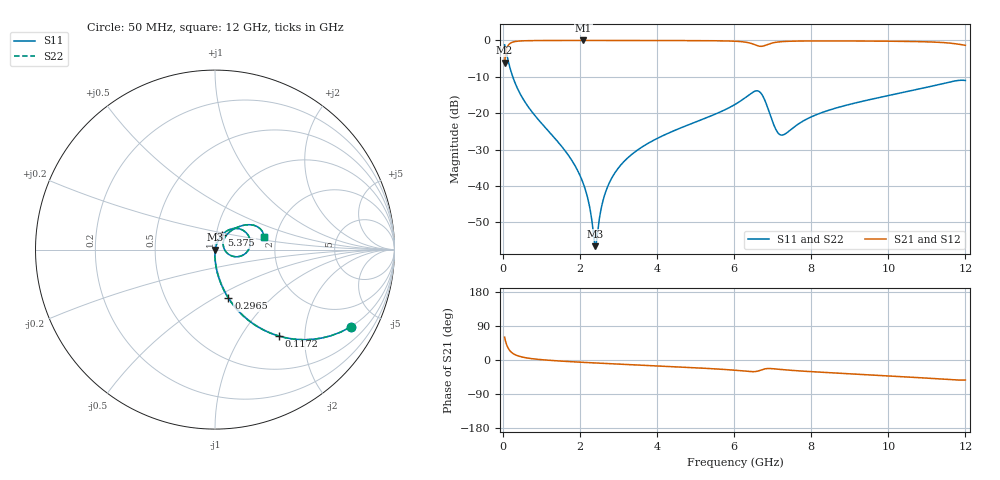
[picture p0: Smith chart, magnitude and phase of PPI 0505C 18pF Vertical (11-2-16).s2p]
# GHz S MA R 50
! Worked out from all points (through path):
!   1601 points, 50 MHz to 12 GHz, reference 50 ohm
!   highest |S21| = -0.01 dB at 2.089 GHz (marker M1); lowest = -6.1 dB at 50 MHz (marker M2)
!   group delay of S21, straight-line fit = 13.9 ps
!   lowest |S11| = -56.6 dB at 2.403 GHz (marker M3), VSWR 1.00, Z = 50.1 - j0.0292 ohm
!   |S11| at or under -10 dB: 261.2 MHz to end of sweep
!   |S22| runs from -56.6 to -1.2 dB; largest |S21 - S12| = 0
!   S11 on the Smith chart (normalised r, x): 50 MHz: 0.99, -3.51; 117.2 MHz: 0.99, -1.49; 296.5 MHz: 0.99, -0.58; 5.375 GHz: 1.07, +0.18; 12 GHz: 1.72, +0.26
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0.05  0.8696 -29.7  0.4937 60.2  0.4937 60.2  0.8696 -29.7
0.1172187  0.5998 -53.5  0.7998 36.5  0.7998 36.5  0.5998 -53.5
0.1919063  0.415 -66.0  0.9094 23.9  0.9094 23.9  0.415 -66.0
0.2964688  0.2809 -74.5  0.9592 15.3  0.9592 15.3  0.2809 -74.5
0.8043438  0.09723 -86.5  0.9943 2.9  0.9943 2.9  0.09723 -86.5
1.655781  0.02858 -91.3  0.9983 -3.8  0.9983 -3.8  0.02858 -91.3
2.044156  0.01243 -89.7  0.9984 -6.0  0.9984 -6.0  0.01243 -89.7
2.088969  0.0108 -88.9  0.9984 -6.2  0.9984 -6.2  0.0108 -88.9
2.230875  0.005913 -83.0  0.9984 -7.0  0.9984 -7.0  0.005913 -83.0
2.402656  0.001482 -11.3  0.9984 -7.8  0.9984 -7.8  0.001482 -11.3
2.626719  0.006985 68.2  0.9983 -9.0  0.9983 -9.0  0.006985 68.2
2.888125  0.01448 73.2  0.9981 -10.3  0.9981 -10.3  0.01448 73.2
3.343719  0.02697 73.7  0.9976 -12.4  0.9976 -12.4  0.02697 73.7
4.038312  0.04576 71.5  0.9965 -15.8  0.9965 -15.8  0.04576 71.5
5.375219  0.09039 64.1  0.9904 -22.6  0.9904 -22.6  0.09039 64.1
6.025  0.1316 55.6  0.9741 -27.0  0.9741 -27.0  0.1316 55.6
6.652375  0.1982 8.2  0.8331 -28.2  0.8331 -28.2  0.1982 8.2
7.085562  0.05952 -8.8  0.9419 -23.7  0.9419 -23.7  0.05952 -8.8
7.227469  0.04991 14.0  0.9603 -25.1  0.9603 -25.1  0.04991 14.0
8.019156  0.08966 51.2  0.9832 -30.8  0.9832 -30.8  0.08966 51.2
10.01331  0.1749 45.1  0.9749 -41.9  0.9749 -41.9  0.1749 45.1
12  0.2811 14.4  0.8563 -52.8  0.8563 -52.8  0.2811 14.4
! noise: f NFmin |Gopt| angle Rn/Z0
0.05  0.0003903  0.8668  1.213  0.0006299
1.372  0.00398  0.6738  4.689  0.002347
2.701  0.006647  0.6271  8.764  0.003321
4.031  0.00959  0.6181  12.81  0.004623
5.36  0.01663  0.6951  17.04  0.01042
6.682  0.1135  0.9368  21.56  0.3867
8.012  0.03143  0.7544  25.52  0.02461
9.341  0.02763  0.6895  29.22  0.01625
10.67  0.03694  0.7311  33.23  0.0252
12  0.1188  0.8981  37.69  0.2283
